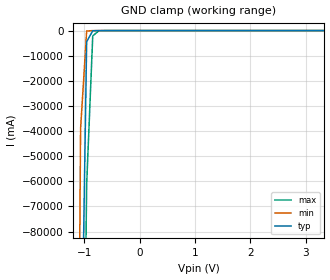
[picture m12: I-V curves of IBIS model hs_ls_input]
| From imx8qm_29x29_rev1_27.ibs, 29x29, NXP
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[Model] hs_ls_input
|   Model hs_ls_input
| This model was characterised for following simulation conditions:
| Spice Models:
|  - Typ Condition
|   /project/usb2_ln28fdsoi/HS/s2ibis/LS_input/ln28fdsoi_lp2.combination ln28fdsoi_typ
|  - Min Condition
|   /project/usb2_ln28fdsoi/HS/s2ibis/LS_input/ln28fdsoi_lp2.combination ln28fdsoi_wcs
|  - Max Condition
|   /project/usb2_ln28fdsoi/HS/s2ibis/LS_input/ln28fdsoi_lp2.combination ln28fdsoi_bcs
Model_type Input
Polarity   Non-Inverting
C_comp   2.8431pF   2.6338pF   3.0727pF
[Temperature Range]   27.0000   -40.0000   0.1050k
[Voltage Range]   3.3000V   3.0000V   3.6000V
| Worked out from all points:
|   GND clamp passes 1 mA (typ) near -0.46 V on its own axis
[GND_clamp]
|Voltage   I(typ)   I(min)   I(max)
-3.6V     -10.68kA   -13.8kA    -8.465kA
-1.18V    -414.1A    -362.8A    -466.3A
-1.07V    -158.9A    -39.07A    -263.8A
-960mV    -4.457A    -179.3mA   -61.22A
-850mV    -76.1mA    -9.541mA   -2.112A
-740mV    -7.894mA   -5.549mA   -83.67mA
3.33V     175.9uA    172.5uA    179uA
